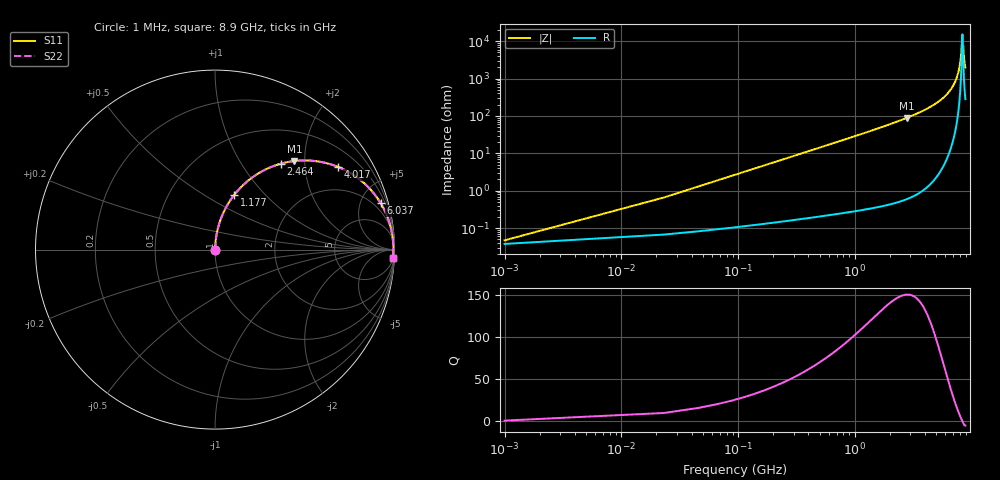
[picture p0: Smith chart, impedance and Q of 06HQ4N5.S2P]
! Coilcraft 0604HQ-4N5 Chip Inductor
! 15 August 2002
# MHZ S MA R 50
!Freq  MagS11  AngS11  MagS21  AngS21  MagS12  AngS12  MagS22  AngS22
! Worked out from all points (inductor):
!   403 points, 1 MHz to 8.9 GHz, reference 50 ohm
!   read as one part in series: L = 4.5 nH near 45.38 MHz
!   highest Q = 150 at 2.797 GHz (marker M1), where L = 5.06 nH
!   self-resonance near 8.389 GHz
!   S11 on the Smith chart (normalised r, x): 1 MHz: 1.00, +0.00; 1.177 GHz: 1.01, +0.68; 2.464 GHz: 1.01, +1.52; 4.017 GHz: 1.02, +2.95; 6.037 GHz: 1.12, +7.08; 8.9 GHz: 7, -39
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1  0.0004711 36.8  0.9996 -0.0  0.9996 -0.0  0.0004711 36.8
67.57  0.01911 86.1  0.9989 -1.1  0.9989 -1.1  0.01911 86.1
134.14  0.03788 86.0  0.9981 -2.2  0.9981 -2.2  0.03788 86.0
222.9  0.06287 85.1  0.9966 -3.6  0.9966 -3.6  0.06287 85.1
378.23  0.1064 82.9  0.9925 -6.1  0.9925 -6.1  0.1064 82.9
577.94  0.1617 79.9  0.9847 -9.3  0.9847 -9.3  0.1617 79.9
1177.07  0.3206 70.8  0.9443 -18.7  0.9443 -18.7  0.3206 70.8
1487.73  0.3972 66.1  0.9145 -23.4  0.9145 -23.4  0.3972 66.1
2464.09  0.6044 52.4  0.7926 -37.2  0.7926 -37.2  0.6044 52.4
2796.94  0.6625 48.1  0.7446 -41.5  0.7446 -41.5  0.6625 48.1
2974.46  0.691 45.9  0.7183 -43.7  0.7183 -43.7  0.691 45.9
4017.39  0.8246 34.0  0.5595 -55.5  0.5595 -55.5  0.8246 34.0
4461.19  0.8662 29.5  0.4925 -60.0  0.4925 -60.0  0.8662 29.5
5947.92  0.9547 16.4  0.2823 -72.7  0.2823 -72.7  0.9547 16.4
6036.68  0.958 15.7  0.2707 -73.3  0.2707 -73.3  0.958 15.7
7434.65  0.9893 5.8  0.1011 -81.0  0.1011 -81.0  0.9893 5.8
7789.69  0.9921 3.6  0.06232 -81.0  0.06232 -81.0  0.9921 3.6
8033.78  0.9932 2.1  0.03675 -78.2  0.03675 -78.2  0.9932 2.1
8189.11  0.9935 1.2  0.02116 -71.4  0.02116 -71.4  0.9935 1.2
8388.82  0.9935 0.0  0.006545 -0.0  0.006545 -0.0  0.9935 0.0
8632.91  0.9929 -1.4  0.02496 72.8  0.02496 72.8  0.9929 -1.4
8900  0.9917 -2.8  0.04999 79.0  0.04999 79.0  0.9917 -2.8
